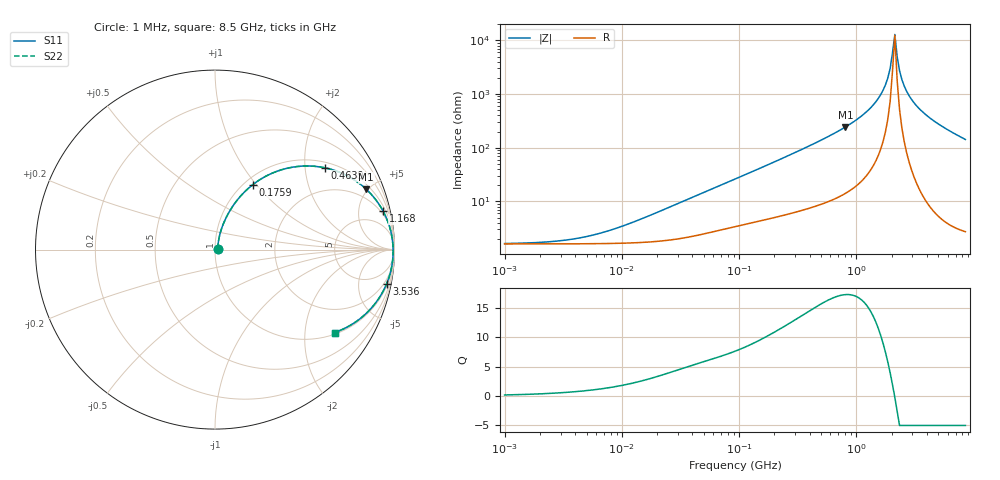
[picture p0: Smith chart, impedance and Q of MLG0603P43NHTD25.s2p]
! S-Parameter Data Generated by TDK Corporation
! Copyright(C) 2025 TDK Corporation.
! All Rights Reserved.
! TDK P/N: MLG0603P43NHTD25 (SMD / SMT Inductor (Coil))
! Property: L=43nH at 300MHz
! Size(LxWxT): 0.6x0.3x0.3mm
! Model Type: s2p (Touchstone File Format Version 1.0)
! Frequency: DC=Yes Start=1MHz Stop=8500MHz 198points Log-sweep
! Model Generated on Feb. 6, 2025
! Terms and conditions regarding TDK Simulation Models:
! 1)This simulation model is being provided solely for informational
!  purposes. Please refer to the specifications of the products in
!  terms of detailed characteristics of such products.
! 2)In no event shall TDK Corporation of any of its subsidiaries be
!  liable for any loss or damage arising, directly or indirectly,
!  from any information contained in this simulation model, including,
!  but not limited to loss or damages arising from any inaccuracies,
!  omissions or errors in connection with such information.
! 3)Any and all copyrights on this simulation model are owned by
!  TDK Corporation.  Duplication or redistribution of this simulation
!  model without prior written permission from TDK Corporation
!  is prohibited.
! 4)This simulation model is subject to any modification or change
!  without any prior notice.
! 5)Neither TDK Corporation nor any of its subsidiaries shall make any
!  warranty, express or implied, including but not limited to the
!  correctness, implied warranties of merchantability and fitness for
!  a particular purpose with respect to this simulation models.
! 6)The use of this simulation model shall be deemed to have consented
!  to the terms and conditions hereof.
! Port Assignments:
!  1 ---@@@--- 2
! Applicable Conditions:
!  Temperature = 25 degC
!  DC Bias Current = 0 A
!  Small Signal Operation
# Hz S MA R 50
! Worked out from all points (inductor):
!   197 points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, 1 MHz to 8.5 GHz, reference 50 ohm
!   read as one part in series: L = 47.4 nH near 18.32 MHz
!   highest Q = 17.3 at 807.2 MHz (marker M1), where L = 48 nH
!   self-resonance near 2.032 GHz
!   S11 on the Smith chart (normalised r, x): 1 MHz: 1.03, +0.01; 175.9 MHz: 1.09, +0.96; 463.9 MHz: 1.17, +2.55; 1.168 GHz: 1.54, +8.59; 3.536 GHz: 1, -10; 8.5 GHz: 1.05, -2.85
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1000000  0.01612 10.4  0.9841 -0.2  0.9841 -0.2  0.01612 10.4
2403882  0.01739 23.7  0.9841 -0.4  0.9841 -0.4  0.01739 23.7
4587603  0.02093 39.6  0.984 -0.8  0.984 -0.8  0.02093 39.6
8755050  0.03051 56.4  0.9835 -1.5  0.9835 -1.5  0.03051 56.4
2.10461e7  0.06401 70.3  0.9803 -3.5  0.9803 -3.5  0.06401 70.3
9.219544e7  0.2444 68.5  0.9384 -14.0  0.9384 -14.0  0.2444 68.5
1.759472e8  0.418 59.8  0.8688 -24.6  0.8688 -24.6  0.418 59.8
4.229561e8  0.7323 39.2  0.6334 -46.9  0.6334 -46.9  0.7323 39.2
4.638648e8  0.7631 36.7  0.5984 -49.6  0.5984 -49.6  0.7631 36.7
8.071757e8  0.907 21.8  0.372 -64.9  0.372 -64.9  0.907 21.8
1.167757e9  0.9608 12.9  0.2233 -73.5  0.2233 -73.5  0.9608 12.9
1.613203e9  0.9852 5.7  0.1006 -78.7  0.1006 -78.7  0.9852 5.7
1.769233e9  0.989 3.8  0.06657 -78.6  0.06657 -78.6  0.989 3.8
1.940355e9  0.9914 1.8  0.03299 -74.0  0.03299 -74.0  0.9914 1.8
2.128028e9  0.9925 -0.1  0.007704 14.7  0.007704 14.7  0.9925 -0.1
2.228565e9  0.9927 -1.1  0.02028 68.2  0.02028 68.2  0.9927 -1.1
2.333852e9  0.9924 -2.1  0.03668 77.1  0.03668 77.1  0.9924 -2.1
2.444114e9  0.9919 -3.0  0.05356 79.8  0.05356 79.8  0.9919 -3.0
2.80715e9  0.9883 -6.0  0.1052 80.6  0.1052 80.6  0.9883 -6.0
3.535948e9  0.9751 -11.2  0.1946 77.1  0.1946 77.1  0.9751 -11.2
5.115526e9  0.9311 -20.3  0.3476 68.6  0.3476 68.6  0.9311 -20.3
8.5e9  0.8109 -34.7  0.5699 54.2  0.5699 54.2  0.8109 -34.7
